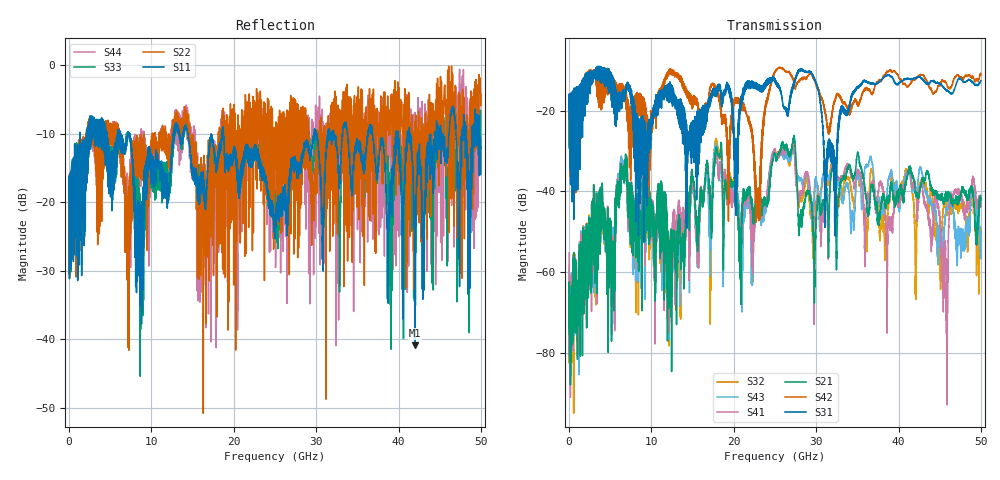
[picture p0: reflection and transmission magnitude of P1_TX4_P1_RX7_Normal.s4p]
!Keysight Technologies,N5225B,MY57041031,A.13.20.10
!Date: Friday, May 31, 2019 11:24:13
!Correction: S11(Full 4 Port(1,2,3,4))
!S12(Full 4 Port(1,2,3,4))
!S13(Full 4 Port(1,2,3,4))
!S14(Full 4 Port(1,2,3,4))
!S21(Full 4 Port(1,2,3,4))
!S22(Full 4 Port(1,2,3,4))
!S23(Full 4 Port(1,2,3,4))
!S24(Full 4 Port(1,2,3,4))
!S31(Full 4 Port(1,2,3,4))
!S32(Full 4 Port(1,2,3,4))
!S33(Full 4 Port(1,2,3,4))
!S34(Full 4 Port(1,2,3,4))
!S41(Full 4 Port(1,2,3,4))
!S42(Full 4 Port(1,2,3,4))
!S43(Full 4 Port(1,2,3,4))
!S44(Full 4 Port(1,2,3,4))
!S4P File: Measurements: <S11,S12,S13,S14>,
!<S21,S22,S23,S24>,
!<S31,S32,S33,S34>,
!<S41,S42,S43,S44>:
# Hz S  dB  R 50.0
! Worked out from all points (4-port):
!   5000 points, 10 MHz to 50 GHz, reference 50 ohm
!   strongest paths, dB at 10 MHz, 12.51 GHz, 25.01 GHz, 37.51 GHz, 50 GHz:
!     S31: -19.7, -17.6, -12.9, -13.1, -12.6
!     S42: -19.5, -9.9, -10.5, -12.8, -11.3
!     S21: -66.4, -57.1, -30.9, -47.2, -42.2
!     S41: -55.2, -50.9, -29.6, -40.3, -43.7
!     S43: -59.5, -52.0, -30.0, -41.4, -51.4
!     S32: -58.2, -58.6, -30.3, -42.2, -50.5
!   lowest |S11| = -40.8 dB at 41.99 GHz (marker M1), VSWR 1.02, Z = 50.9 - j0.146 ohm
!   |S11| at or under -10 dB: 7.336 GHz to 12.7 GHz (5.362 GHz wide, 53.5 % of centre); 14.41 GHz to 18.57 GHz (4.157 GHz wide, 25.2 % of centre); 18.74 GHz to 29.76 GHz (11.02 GHz wide, 45.4 % of centre)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
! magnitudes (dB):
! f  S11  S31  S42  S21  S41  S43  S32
! 10 MHz  -19.4  -19.7  -19.5  -66.4  -55.2  -59.5  -58.2
! 6.41 GHz  -11.7  -18.5  -15.3  -34.9  -34.3  -33.0  -33.2
! 17.88 GHz  -14.7  -14.7  -15.0  -28.9  -30.2  -28.5  -26.9
! 22.93 GHz  -13.3  -14.8  -39.5  -40.0  -41.2  -40.4  -40.9
! 25.28 GHz  -21.4  -13.2  -9.6  -31.5  -31.1  -30.7  -30.9
! 41.99 GHz  -40.8  -12.0  -12.3  -39.2  -37.5  -38.6  -49.5
! 50 GHz  -12.0  -12.6  -11.3  -42.2  -43.7  -51.4  -50.5
